| IBIS file rt600_bga176_dr2.ibs generated by Viper version: 2020.03.08
[IBIS Ver]   5.0
[Comment Char]   |_char
[File Name]   rt600_bga176_dr2.ibs
[File Rev]   1.3
[Date]   Sun Mar  8 20:14:53 2020
[Source]   NXP Viper 2020.03.08
[Notes]
[Disclaimer] IMPORTANT NOTICE
  This information is provided on an AS IS basis and without warranty.
  IN NO EVENT SHALL NXP BE LIABLE FOR INCIDENTAL OR CONSEQUENTIAL
  DAMAGES ARISING FROM USE OF THIS INFORMATION. THIS DISCLAIMER OF
  WARRANTY EXTENDS TO THE USER OF THE INFORMATION, AND TO THEIR CUSTOMERS
  OR USERS OF PRODUCTS  AND IS IN LIEU OF ALL WARRANTIES WHETHER EXPRESS,
  IMPLIED, OR STATUTORY, INCLUDING IMPLIED WARRANTIES OF MERCHANTABILITY
  OR FITNESS FOR PARTICULAR PURPOSE.
  NXP does not represent or warrant that the information furnished
  hereunder is free of infringement of any third party patents,
  copyrights, trade secrets, or other intellectual property rights.
  NXP does not represent or warrant that the information is free of
  defect, or that it meets any particular standard, requirements or need
  of the user of the infomation or their customers.
  NXP reserves the right to change the information in this file
  without notice.
   http://www.nxp.com
[Copyright]   (C) Copyright NXP 2004 - 2020, All Rights Reserved.
|   BGA176
[Component]   BGA176
[Manufacturer]   NXP
[Package]
| variable   typ   min   max
R_pkg   0.14129   0.09613   0.19985
L_pkg   2.273e-09   1.470e-09   3.459e-09
C_pkg   3.279e-13   2.049e-13   4.953e-13
[Pin] signal_name   model_name   R_pin   L_pin   C_pin
A1   PIO0_19   gpio   0.19985   3.360e-09 4.051e-13
A2   PIO0_26   gpio   0.18441   3.042e-09 4.517e-13
A3   PIO0_14   gpio   0.15295   2.662e-09 3.035e-13
A5   PIO0_15   gpio   0.13033   2.093e-09 2.697e-13
A7   PIO1_2   gpio   0.15052   2.097e-09 3.235e-13
A9   PIO0_25   gpio   0.1235   1.937e-09 2.898e-13
A11   PIO0_31   gpio   0.12513   2.036e-09 2.648e-13
A13   VDD_FUSE18   POWER   NA   NA   NA
A15   INTN   gpio   0.16043   2.544e-09 3.436e-13
A16   LDO_ENABLE   gpio   0.1535   2.759e-09 3.410e-13
A17   XTALOUT32KHZ   NC   0.15193   2.784e-09 3.881e-13
B1   PIO1_9   gpio   0.17844   3.238e-09 3.024e-13
B2   PIO0_20   gpio   0.17097   2.590e-09 3.870e-13
B3   PIO0_27   gpio   0.14332   1.901e-09 3.520e-13
B5   PIO1_8   gpio   0.16351   2.692e-09 3.404e-13
B6   PIO2_31   gpio   0.15828   2.326e-09 2.666e-13
B7   PIO0_18   gpio   0.11019   1.671e-09 3.015e-13
B9   PIO0_24   gpio   0.10819   1.627e-09 2.930e-13
B10   PIO0_29   gpio   0.13962   2.165e-09 2.904e-13
B11   VDD_PLL18   POWER   NA   NA   NA
B13   XTALOUTSYS   NC   0.17111   2.970e-09 3.988e-13
B14   XTALINSYS   NC   0.17378   2.931e-09 4.149e-13
B15   RESETN   gpio   0.14511   2.256e-09 3.603e-13
B16   PMIC_MODE1   reset   0.13243   2.317e-09 3.355e-13
B17   XTALIN32KHZ   NC   0.15731   2.811e-09 3.707e-13
C1   PIO2_14   gpio   0.14605   2.368e-09 2.923e-13
C2   VREFL_ANA   NC   0.14411   2.079e-09 2.646e-13
C3   VSS_ADC_ANA   GND   NA   NA   NA
C4   VDD33_ADC_ANA   POWER   NA   NA   NA
C5   VDDCORE_CAP   POWER   NA   NA   NA
C7   PIO0_21   gpio   0.10988   1.606e-09 3.544e-13
C9   PIO0_23   gpio   0.11115   1.626e-09 3.596e-13
C11   PIO0_30   gpio   0.14728   2.482e-09 3.186e-13
C13   VDD_AO18   POWER   NA   NA   NA
C15   PMIC_MODE0   reset   0.10232   1.617e-09 3.963e-13
C16   VDD1V8_DRV   POWER   NA   NA   NA
C17   VDD1V8_DRV   POWER   NA   NA   NA
D2   VREFH_ANA18   NC   0.13705   1.862e-09 3.088e-13
D5   GND   GND   NA   NA   NA
D6   PIO0_16   gpio   0.16446   2.830e-09 3.433e-13
D7   PIO0_17   gpio   0.12939   2.060e-09 3.801e-13
D8   PIO0_22   gpio   0.11253   1.654e-09 3.709e-13
D9   VDDCORE_CAP   POWER   NA   NA   NA
D11   PIO0_28   gpio   0.16253   2.726e-09 3.499e-13
D12   GND   GND   NA   NA   NA
D13   VDDEAO   POWER   NA   NA   NA
D15   GND   GND   NA   NA   NA
E1   PIO0_6   gpio   0.12421   1.791e-09 2.705e-13
E2   PIO2_15   gpio   0.13427   1.840e-09 2.726e-13
E3   PIO0_12   gpio   0.13877   2.137e-09 3.324e-13
E4   VDD18_ADC_ANA   POWER   NA   NA   NA
E6   VDDE1   POWER   NA   NA   NA
E8   VDDE1   POWER   NA   NA   NA
E10   VDDE1   POWER   NA   NA   NA
E12   GND   GND   NA   NA   NA
E14   GND   GND   NA   NA   NA
E15   VDD1V8_DRV   POWER   NA   NA   NA
E16   FC15_SCL   gpio   0.15171   2.261e-09 3.659e-13
E17   PIO1_0   gpio   0.14604   2.360e-09 2.754e-13
F4   PIO0_5   gpio   0.13449   1.997e-09 3.676e-13
F5   VDDE0   POWER   NA   NA   NA
F7   GND   GND   NA   NA   NA
F11   GND   GND   NA   NA   NA
F13   VDD1V8   POWER   NA   NA   NA
F14   VDDCORE_CAP   POWER   NA   NA   NA
F16   FC15_SDA   gpio   0.13227   1.997e-09 3.189e-13
G1   PIO0_0   gpio   0.12567   1.994e-09 2.049e-13
G2   PIO0_1   gpio   0.14405   2.372e-09 2.631e-13
G3   PIO0_13   gpio   0.12919   2.036e-09 3.436e-13
G4   PIO0_2   gpio   0.16644   2.693e-09 4.122e-13
G6   GND   GND   NA   NA   NA
G12   GND   GND   NA   NA   NA
G14   VDD18_IOREF_1   POWER   NA   NA   NA
G15   PIO1_1   gpio   0.16428   2.686e-09 3.296e-13
G16   PIO1_3   gpio   0.1231   1.714e-09 2.821e-13
G17   PIO1_4   gpio   0.13341   2.155e-09 2.558e-13
H2   PIO0_3   gpio   0.1129   1.749e-09 2.771e-13
H5   VDDE0   POWER   NA   NA   NA
H8   GND   GND   NA   NA   NA
H9   GND   GND   NA   NA   NA
H10   GND   GND   NA   NA   NA
H13   VDDE1   POWER   NA   NA   NA
H14   VDDE1   POWER   NA   NA   NA
J1   PIO0_4   gpio   0.12668   2.038e-09 2.695e-13
J2   PIO0_7   gpio   0.14281   2.387e-09 2.733e-13
J3   PIO0_10   gpio   0.10827   1.614e-09 3.750e-13
J4   VDDCORE_CAP   POWER   NA   NA   NA
J8   GND   GND   NA   NA   NA
J10   GND   GND   NA   NA   NA
J14   VDDCORE_CAP   POWER   NA   NA   NA
J15   PIO1_7   gpio   0.15476   2.446e-09 3.371e-13
J16   PIO1_5   gpio   0.11365   1.766e-09 2.497e-13
J17   PIO1_6   gpio   0.12517   2.022e-09 2.737e-13
K4   PIO0_8   gpio   0.16241   2.729e-09 3.960e-13
K5   VDDE0   POWER   NA   NA   NA
K8   GND   GND   NA   NA   NA
K9   GND   GND   NA   NA   NA
K10   GND   GND   NA   NA   NA
K13   VDDE1   POWER   NA   NA   NA
K16   PIO1_10   gpio   0.11938   1.877e-09 2.863e-13
L1   PIO0_11   gpio   0.13639   2.262e-09 3.272e-13
L2   PIO1_11   gpio   0.1447   2.390e-09 3.502e-13
L3   PIO0_9   gpio   0.16352   2.908e-09 4.164e-13
L4   VDD18_IOREF_0   POWER   NA   NA   NA
L6   GND   GND   NA   NA   NA
L12   GND   GND   NA   NA   NA
L14   VDDE1   POWER   NA   NA   NA
L15   PIO2_26   gpio   0.10997   1.567e-09 3.422e-13
L16   PIO2_24   gpio   0.11574   1.651e-09 2.912e-13
L17   PIO2_25   gpio   0.12638   2.020e-09 2.817e-13
M2   PIO1_12   gpio   0.15125   2.660e-09 3.053e-13
M4   PIO1_16   gpio   0.1256   1.772e-09 4.884e-13
M5   VDDE0   POWER   NA   NA   NA
M7   GND   GND   NA   NA   NA
M11   GND   GND   NA   NA   NA
M13   GND   GND   NA   NA   NA
M14   PIO2_27   gpio   0.17483   3.019e-09 4.180e-13
N1   PIO1_13   gpio   0.15598   2.607e-09 3.370e-13
N2   PIO1_14   gpio   0.17372   3.138e-09 3.860e-13
N3   PIO1_15   gpio   0.19064   3.248e-09 4.953e-13
N4   PIO1_17   gpio   0.18718   3.167e-09 4.589e-13
N6   VDDE0   POWER   NA   NA   NA
N8   VDDE0   POWER   NA   NA   NA
N10   VDDE0   POWER   NA   NA   NA
N12   VDDE2   POWER   NA   NA   NA
N14   GND   GND   NA   NA   NA
N15   PIO2_28   gpio   0.14645   2.334e-09 3.746e-13
N16   VDD_USB33   POWER   NA   NA   NA
N17   PIO2_29   gpio   0.12481   1.949e-09 2.239e-13
P3   PIO2_22   gpio   0.09613   1.552e-09 3.927e-13
P5   PIO2_23   gpio   0.10263   1.740e-09 4.243e-13
P6   PIO1_22   sd_mmc   0.15046   2.295e-09 3.313e-13
P7   PIO1_23   sd_mmc   0.16934   2.938e-09 3.792e-13
P9   VDDCORE_CAP   POWER   NA   NA   NA
P10   PIO1_30   sd_mmc   0.11625   1.636e-09 3.115e-13
P11   VDDE2   POWER   NA   NA   NA
P12   VDDE2   POWER   NA   NA   NA
P13   GND   GND   NA   NA   NA
P16   PIO2_30   gpio   0.12795   2.102e-09 2.091e-13
R1   PIO2_16   gpio   0.16913   2.881e-09 3.340e-13
R2   PIO2_18   gpio   0.15178   2.328e-09 3.897e-13
R3   PIO2_21   gpio   0.11283   1.794e-09 3.660e-13
R5   VDDCORE_CAP   POWER   NA   NA   NA
R7   PIO1_26   sd_mmc   0.12201   1.824e-09 2.999e-13
R9   PIO1_31   sd_mmc   0.13786   1.914e-09 2.941e-13
R11   PIO2_0   sd_mmc   0.14159   2.111e-09 2.534e-13
R13   PIO2_9   gpio   0.10419   1.762e-09 3.011e-13
R14   VDDCORE_CAP   POWER   NA   NA   NA
R15   VDD_USB18   POWER   NA   NA   NA
R16   USB0_VBUS_DETECT   NC   0.14096   2.222e-09 2.560e-13
R17   USB0_DP   NC   0.15874   2.505e-09 2.940e-13
T1   PIO2_13   gpio   0.18034   3.170e-09 4.238e-13
T2   PIO2_19   gpio   0.15149   2.497e-09 3.868e-13
T3   PIO2_12   gpio   0.12679   1.923e-09 3.321e-13
T4   PIO1_19   sd_mmc   0.13088   2.075e-09 3.021e-13
T5   PIO1_20   sd_mmc   0.12113   1.945e-09 3.088e-13
T7   PIO1_24   sd_mmc   0.13518   2.351e-09 2.896e-13
T8   PIO1_27   sd_mmc   0.11249   1.792e-09 2.593e-13
T9   PIO1_18   sd_mmc   0.10662   1.470e-09 2.234e-13
T11   PIO2_1   sd_mmc   0.14569   2.205e-09 2.732e-13
T12   PIO2_3   sd_mmc   0.13739   1.902e-09 2.414e-13
T13   PIO2_4   sd_mmc   0.15111   2.320e-09 3.303e-13
T15   PIO2_10   gpio   0.098335  1.592e-09 2.753e-13
T16   PIO2_11   gpio   0.15817   2.622e-09 4.285e-13
T17   USB0_DM   NC   0.16291   2.699e-09 2.840e-13
U1   PIO2_17   gpio   0.19357   3.459e-09 4.074e-13
U2   PIO2_20   gpio   0.14297   2.419e-09 3.756e-13
U3   PIO1_29   sd_mmc   0.13825   2.359e-09 3.429e-13
U5   PIO1_21   sd_mmc   0.13241   2.209e-09 2.751e-13
U7   PIO1_25   sd_mmc   0.12302   1.980e-09 2.361e-13
U9   PIO1_28   sd_mmc   0.12084   1.946e-09 2.552e-13
U11   PIO2_2   sd_mmc   0.12253   1.925e-09 2.360e-13
U13   PIO2_5   sd_mmc   0.14796   2.223e-09 2.730e-13
U15   PIO2_6   sd_mmc   0.14325   2.512e-09 3.357e-13
U16   PIO2_7   sd_mmc   0.1746   3.003e-09 3.709e-13
U17   PIO2_8   sd_mmc   0.17231   3.255e-09 3.576e-13
[Pin Mapping]   pulldown_ref   pullup_ref
A1   GND   VDDE1
A2   GND   VDDE1
A3   GND   VDDE1
A5   GND   VDDE1
A7   GND   VDDE1
A9   GND   VDDE1
A11   GND   VDDE1
A13   NC   VDD_FUSE18
A15   GND   VDDEAO
A16   GND   VDDEAO
A17   NC   NC
B1   GND   VDDE1
B2   GND   VDDE1
B3   GND   VDDE1
B5   GND   VDDE1
B6   GND   VDDE1
B7   GND   VDDE1
B9   GND   VDDE1
B10   GND   VDDE1
B11   NC   VDD_PLL18
B13   NC   NC
B14   NC   NC
B15   GND   VDDEAO
B16   GND   VDDEAO
B17   NC   NC
C1   GND   VDDE0
C2   NC   NC
C3   VSS_ADC_ANA   NC
C4   NC   VDD33_ADC_ANA
C5   NC   VDDCORE_CAP
C7   GND   VDDE1
C9   GND   VDDE1
C11   GND   VDDE1
C13   NC   VDD_AO18
C15   GND   VDDEAO
C16   NC   VDD1V8_DRV
C17   NC   VDD1V8_DRV
D2   NC   NC
D5   GND   NC
D6   GND   VDDE1
D7   GND   VDDE1
D8   GND   VDDE1
D9   NC   VDDCORE_CAP
D11   GND   VDDE1
D12   GND   NC
D13   NC   VDDEAO
D15   GND   NC
E1   GND   VDDE0
E2   GND   VDDE0
E3   GND   VDDE0
E4   NC   VDD18_ADC_ANA
E6   NC   VDDE1
E8   NC   VDDE1
E10   NC   VDDE1
E12   GND   NC
E14   GND   NC
E15   NC   VDD1V8_DRV
E16   GND   VDDE1
E17   GND   VDDE1
F4   GND   VDDE0
F5   NC   VDDE0
F7   GND   NC
F11   GND   NC
F13   NC   VDD1V8
F14   NC   VDDCORE_CAP
F16   GND   VDDE1
G1   GND   VDDE0
G2   GND   VDDE0
G3   GND   VDDE0
G4   GND   VDDE0
G6   GND   NC
G12   GND   NC
G14   NC   VDD18_IOREF_1
G15   GND   VDDE1
G16   GND   VDDE1
G17   GND   VDDE1
H2   GND   VDDE0
H5   NC   VDDE0
H8   GND   NC
H9   GND   NC
H10   GND   NC
H13   NC   VDDE1
H14   NC   VDDE1
J1   GND   VDDE0
J2   GND   VDDE0
J3   GND   VDDE0
J4   NC   VDDCORE_CAP
J8   GND   NC
J10   GND   NC
J14   NC   VDDCORE_CAP
J15   GND   VDDE1
J16   GND   VDDE1
J17   GND   VDDE1
K4   GND   VDDE0
K5   NC   VDDE0
K8   GND   NC
K9   GND   NC
K10   GND   NC
K13   NC   VDDE1
K16   GND   VDDE1
L1   GND   VDDE0
L2   GND   VDDE0
L3   GND   VDDE0
L4   NC   VDD18_IOREF_0
L6   GND   NC
L12   GND   NC
L14   NC   VDDE1
L15   GND   VDDE1
L16   GND   VDDE1
L17   GND   VDDE1
M2   GND   VDDE0
M4   GND   VDDE0
M5   NC   VDDE0
M7   GND   NC
M11   GND   NC
M13   GND   NC
M14   GND   VDDE1
N1   GND   VDDE0
N2   GND   VDDE0
N3   GND   VDDE0
N4   GND   VDDE0
N6   NC   VDDE0
N8   NC   VDDE0
N10   NC   VDDE0
N12   NC   VDDE2
N14   GND   NC
N15   GND   VDDE1
N16   NC   VDD_USB33
N17   GND   VDDE1
P3   GND   VDDE0
P5   GND   VDDE0
P6   GND   VDDE0
P7   GND   VDDE0
P9   NC   VDDCORE_CAP
P10   GND   VDDE2
P11   NC   VDDE2
P12   NC   VDDE2
P13   GND   NC
P16   GND   VDDE1
R1   GND   VDDE0
R2   GND   VDDE0
R3   GND   VDDE0
R5   NC   VDDCORE_CAP
R7   GND   VDDE0
R9   GND   VDDE2
R11   GND   VDDE2
R13   GND   VDDE2
R14   NC   VDDCORE_CAP
R15   NC   VDD_USB18
R16   NC   NC
R17   NC   NC
T1   GND   VDDE0
T2   GND   VDDE0
T3   GND   VDDE0
T4   GND   VDDE0
T5   GND   VDDE0
T7   GND   VDDE0
T8   GND   VDDE0
T9   GND   VDDE0
T11   GND   VDDE2
T12   GND   VDDE2
T13   GND   VDDE2
T15   GND   VDDE2
T16   GND   VDDE2
T17   NC   NC
U1   GND   VDDE0
U2   GND   VDDE0
U3   GND   VDDE0
U5   GND   VDDE0
U7   GND   VDDE0
U9   GND   VDDE0
U11   GND   VDDE2
U13   GND   VDDE2
U15   GND   VDDE2
U16   GND   VDDE2
U17   GND   VDDE2
|*   Model Selector   *
[Model Selector] gpio
io_obe1dse0sre0   5mA current driving capability, without slew rate
io_obe1dse0sre1   5mA current driving capability, with slew rate
io_obe1dse1sre0   10mA current driving capability, without slew rate
io_obe1dse1sre1   10mA current driving capability, with slew rate
[Model Selector] reset
io_rst_obe1dse0sre0   5mA current driving capability, without slew rate
io_rst_obe1dse0sre1   5mA current driving capability, with slew rate
io_rst_obe1dse1sre0   10mA current driving capability, without slew rate
io_rst_obe1dse1sre1   10mA current driving capability, with slew rate
[Model Selector] sd_mmc
BDPROGSCARUDQP_SDMMC_3V3SF_00_SD   PSW=0 PDRV=0 MODE=1V8 SD
BDPROGSCARUDQP_SDMMC_3V3SF_01_SD   PSW=0 PDRV=1 MODE=1V8 SD
BDPROGSCARUDQP_SDMMC_3V3SF_00_MMC   PSW=0 PDRV=0 MODE=1V8 MMC
BDPROGSCARUDQP_SDMMC_3V3SF_01_MMC   PSW=0 PDRV=1 MODE=1V8 MMC
BDPROGSCARUDQP_SDMMC_3V3SF_10   PSW=1 PDRV=0 MODE=3V3 SD & 3V3 MMC
BDPROGSCARUDQP_SDMMC_3V3SF_11   PSW=1 PDRV=1 MODE=3V3 SD & 3V3 MMC
BDPROGSCARUDQP_SDMMC_3V3SF_11_2v7   PSW=1 PDRV=1 MODE=2V7 SD & 2V7 MMC
BDPROGSCARUDQP_SDMMC_3V3SF_10_2v7   PSW=1 PDRV=0 MODE=2V7 SD & 2V7 MMC
| End [Component] BGA176
| Models and submodels in the file (16): BDPROGSCARUDQP_SDMMC_3V3SF_00_MMC (I/O), BDPROGSCARUDQP_SDMMC_3V3SF_00_SD (I/O), BDPROGSCARUDQP_SDMMC_3V3SF_01_MMC (I/O), BDPROGSCARUDQP_SDMMC_3V3SF_01_SD (I/O), BDPROGSCARUDQP_SDMMC_3V3SF_10 (I/O), BDPROGSCARUDQP_SDMMC_3V3SF_10_2v7 (I/O), BDPROGSCARUDQP_SDMMC_3V3SF_11 (I/O), BDPROGSCARUDQP_SDMMC_3V3SF_11_2v7 (I/O), io_obe1dse0sre0 (I/O), io_obe1dse0sre1 (I/O), io_obe1dse1sre0 (I/O), io_obe1dse1sre1 (I/O), io_rst_obe1dse0sre0 (I/O), io_rst_obe1dse0sre1 (I/O), io_rst_obe1dse1sre0 (I/O), io_rst_obe1dse1sre1 (I/O)
